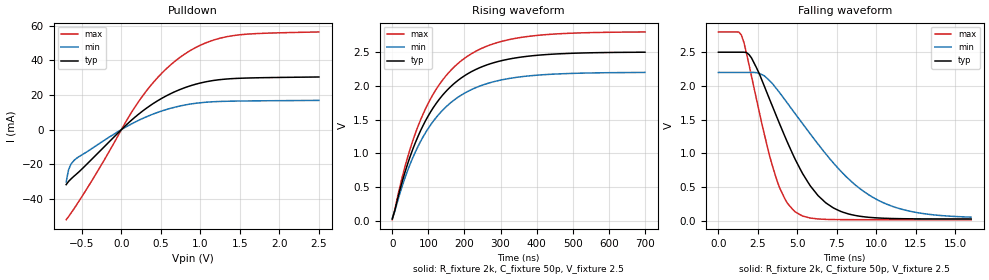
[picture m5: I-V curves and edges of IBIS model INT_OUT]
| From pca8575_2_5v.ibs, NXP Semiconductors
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[Model]   INT_OUT
Model_type Open_drain
Vref=2.5
Vmeas=1.25
Rref=2k
Cref=50p
C_comp   5.4p   5.2p   5.7p
[Temperature Range] 27   85   -40
[Voltage Range]   2.5   2.2   2.8
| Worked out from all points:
|   slope of the pulldown table from 0 to 0.375 V, typ, clamps not added: 26.4 ohm
|   falling waveform, R_fixture 2k, C_fixture 50p, V_fixture 2.5: 20-80 % time 2.92ns typ, 4.64ns min, 1.74ns max; typ from 2.5 V to 0.028 V
|   rising waveform, R_fixture 2k, C_fixture 50p, V_fixture 2.5: 20-80 % time 141ns typ, 141ns min, 140ns max; typ from 0.028 V to 2.5 V
[Pulldown]
-700mV    -31.75mA   -30.26mA   -51.97mA
-670mV    -29.91mA   -23.23mA   -50.18mA
-640mV    -28.51mA   -19.97mA   -48.29mA
-540mV    -24.45mA   -15.68mA   -41.44mA
80mV      3.487mA    2.092mA    6.367mA
240mV     9.708mA    5.82mA     17.62mA
460mV     16.67mA    9.945mA    30.08mA
720mV     22.71mA    13.39mA    40.93mA
1.01V     26.98mA    15.53mA    48.88mA
1.34V     29.2mA     16.34mA    53.62mA
1.69V     29.85mA    16.57mA    55.32mA
2.5V      30.34mA    16.83mA    56.3mA
[Falling Waveform]
R_fixture=2k
C_fixture=50p
V_fixture=2.5
V_fixture_min=2.2
V_fixture_max=2.8
0s        2.5V       2.2V       2.8V
1.455ns   2.5V       2.2V       2.754V
2.101ns   2.413V     2.2V       2.139V
3.394ns   1.713V     2.042V     833.6mV
4.202ns   1.255V     1.797V     328.5mV
4.848ns   918mV      1.592V     135.2mV
6.788ns   269mV      996mV      21.82mV
9.697ns   48.97mV    359.5mV    17.03mV
12.12ns   30.32mV    142.5mV    16.99mV
16ns      27.84mV    54.84mV    16.99mV
[Rising Waveform]
R_fixture=2k
C_fixture=50p
V_fixture=2.5
V_fixture_min=2.2
V_fixture_max=2.8
0s        27.75mV    40.61mV    16.99mV
21.21ns   458.5mV    407.5mV    509.7mV
42.42ns   842.2mV    743.6mV    941.1mV
63.64ns   1.154V     1.017V     1.292V
84.85ns   1.408V     1.239V     1.576V
134.3ns   1.829V     1.609V     2.049V
198ns     2.141V     1.884V     2.399V
268.7ns   2.321V     2.042V     2.601V
360.6ns   2.428V     2.136V     2.72V
700ns     2.497V     2.198V     2.797V
[Ramp]
R_load=2k
dV/dt_r   1.962E+0/2.292E-9   1.952E+0/2.527E-9   1.970E+0/2.035E-9
dV/dt_f   1.962E+0/1.351E-10   1.953E+0/2.447E-10   1.970E+0/7.871E-11
|[End   INT_OUT
